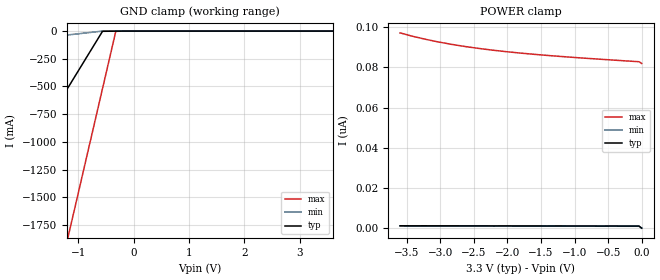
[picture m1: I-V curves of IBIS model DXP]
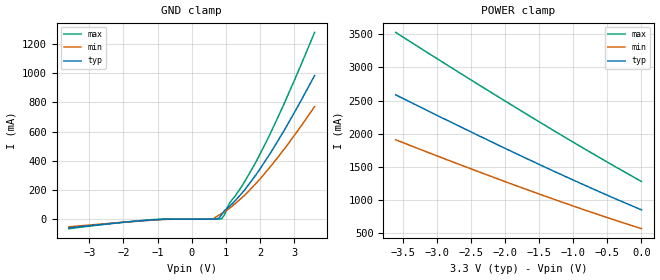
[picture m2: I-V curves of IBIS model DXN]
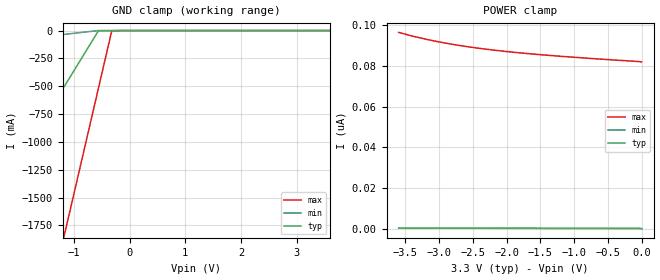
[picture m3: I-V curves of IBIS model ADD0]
| IBIS file MAX6654.ibs created at Maxim Integrated Products
[IBIS ver]   3.2
[File name]   max6654.ibs
[File Rev]   1.0
[Date]   February 19, 2010
[Source]   Data was acquired from HSpice simulations.
[Notes]   This is a microprocessor voltage monitor.
[Disclaimer] Maxim Integrated Products hereby grants the user of this
   IBIS model a non-exclusive, nontransferable license to use
   this IBIS model under the following terms. Before using
   this IBIS model, the user should read this license. If the
   user does not accept these terms, the IBIS model should be
   returned to Maxim Integrated Products within 30 days.
   The user is granted this license only to use the IBIS model
   and is not granted rights to sell, load, rent, lease or
   license the IBIS model in whole or in part, or in modified
   form to anyone other than user. User may modify the IBIS
   model to suit its specific applications but rights to
   derivative works and such modifications shall belong to
   Maxim Integrated Products. This IBIS model is provided on
   an "AS IS" basis and Maxim Integrated Products makes
   absolutely no warranty with respect to the information
   contained herein.MAXIM INTEGRATED PRODUCTS DISCLAIMS AND
   CUSTOMER WAIVES ALL WARRANTIES, EXPRESS OR IMPLIED,
   INCLUDING WARRANTIES OF MERCHANTABILITY OR FITNESS FOR A
   PARTICULAR PURPOSE. The entire risk as to quality and
   performance is with the Customer. ACCORDINGLY, IN NO EVENT
   SHALL THE COMPANY BE LIABLE FOR ANY DAMAGES, WHETHER IN
   CONTRACT OR TORT,INCLUDING ANY LOST PROFITS OR OTHER
   INCIDENTAL, CONSEQUENTIAL, EXEMPLARY, OR PUNITIVE DAMAGES
   ARISING OUT OF THE USE OR APPLICATION OF THE IBIS model
   provided in this package.Further, Maxim Integrated Products
   reserves the right to make changes without notice to any
   product herein to improve reliability, function, or design.
   Maxim Integrated Products does not convey any license under
   patent rights or any other intellectual property rights,
   including those of third parties.
   Maxim Integrated Products is not obligated to provide
   maintenance or support for the licensed IBIS model.
[Copyright]   Copyright of Maxim Integrated Products.
|   Component MAX6654
[Component]   MAX6654
[Manufacturer]   Maxim Integrated Products
[Package]
|variable   typ   min   max
R_pkg   0.052ohm   0.041ohm   0.065ohm
L_pkg   1.440nH   1.005nH   1.870nH
C_pkg   0.222pF   0.164pF   0.271pF
[Pin]  signal_name   model_name   R_pin   L_pin   C_pin
1   N.C   NC   NA   NA   NA
2   VCC   POWER   0.052   1.440nH   0.222pF
3   DXP   DXP   0.052   1.440nH   0.222pF
4   DXN   DXN   0.041   1.005nH   0.164pF
5   N.C   NC   NA   NA   NA
6   ADD1   ADD1   0.052   1.440nH   0.222pF
7   GND   GND   0.052   1.440nH   0.222pF
8   GND   GND   0.065   1.870nH   0.271pF
9   N.C   NC   NA   NA   NA
10   ADD0   ADD0   0.052   1.440nH   0.222pF
11   /ALERT\   ALERTB   0.052   1.440nH   0.222pF
12   SMBDATA   SMBDATA   0.041   1.005nH   0.164pF
13   N.C   NC   NA   NA   NA
14   SMBCLK   SMBCLK   0.052   1.440nH   0.222pF
15   /STBY\   STBYB   0.052   1.440nH   0.222pF
16   N.C   NC   NA   NA   NA
| Models and submodels in the file (8): DXP (Terminator), DXN (Terminator), ADD0 (Input), ADD1 (Input), SMBCLK (Input), STBYB (Input), ALERTB (Open_drain), SMBDATA (I/O_open_drain)
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|   DXP Input
[Model]   DXP
|Signals   DXP
Model_type   Terminator
C_comp   3.195E-12   2.653E-12   3.683E-12
[Temperature Range]   25   -55   125
[Voltage Range]   3.30V   3.00V   3.60V
[Pullup Reference]   3.30V   3.00V   3.60V
[Pulldown Reference]   0.00V   0.00V   0.00V
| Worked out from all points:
|   GND clamp passes 1 mA (typ) near -0.37 V on its own axis
[POWER_clamp]
| Note that the [POWER_clamp] voltage table is referenced to Vcc
| and is calculated using Vtable=Vcc - Vmeasured.
|V(V)   I(typ)   I(min)   I(max)
-3.6V     1.302nA    1.18nA     97.03nA
-3.4V     1.279nA    1.164nA    95.26nA
-3.24V    1.288nA    1.165nA    94.01nA
-3.04V    1.265nA    1.15nA     92.61nA
-2.84V    1.273nA    1.15nA     91.39nA
-2.72V    1.261nA    1.142nA    90.74nA
-2.36V    1.252nA    1.13nA     89.03nA
-2V       1.244nA    1.119nA    87.65nA
-1.44V    1.205nA    1.09nA     85.94nA
-840mV    1.206nA    1.077nA    84.46nA
-40mV     1.168nA    1.045nA    82.72nA
0V        129pA      112.7pA    81.88nA
[GND_clamp]
| Note that the [GND_clamp] voltage table is referenced to Gnd.
|V(V)   I(typ)   I(min)   I(max)
-3.6V     -2.483A    -169.4mA   -7.066A
-2.8V     -1.83A     -124.8mA   -5.343A
-2.72V    -1.765A    -120.3mA   -5.171A
-1.2V     -524.3mA   -35.66mA   -1.897A
-1.12V    -459mA     -31.2mA    -1.725A
-560mV    -1.93mA    -1.782uA   -519.1mA
-320mV    -772.1uA   -711.6nA   -2.201mA
3.6V      2.468nA    2.184nA    83.49nA
|   DXN Input
[Model]   DXN
|Signals   DXN
Model_type   Terminator
C_comp   0.484E-09   0.353E-09   0.676E-09
[Temperature Range]   25   -55   125
[Voltage Range]   3.30V   3.00V   3.60V
[Pullup Reference]   3.30V   3.00V   3.60V
[Pulldown Reference]   0.00V   0.00V   0.00V
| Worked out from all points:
|   GND clamp passes 1 mA (typ) near -0.79 V on its own axis
[POWER_clamp]
| Note that the [POWER_clamp] voltage table is referenced to Vcc
| and is calculated using Vtable=Vcc - Vmeasured.
|V(V)   I(typ)   I(min)   I(max)
-3.6V     2.586A     1.909A     3.525A
-2.64V    2.099A     1.527A     2.901A
-1.68V    1.625A     1.16A      2.293A
-920mV    1.266A     883.7mA    1.824A
0V        854mA      571.2mA    1.281A
[GND_clamp]
| Note that the [GND_clamp] voltage table is referenced to Gnd.
|V(V)   I(typ)   I(min)   I(max)
-3.6V     -60.67mA   -53.22mA   -65.81mA
-1.2V     -6.363mA   -8.032mA   -4.655mA
560mV     5.91uA     780.7uA    89.3uA
800mV     6.397mA    27.47mA    263.9uA
880mV     31.11mA    38.11mA    2.348mA
960mV     57.88mA    49.7mA     28.97mA
1.12V     90.13mA    76.22mA    114.1mA
1.52V     190.7mA    157.1mA    245mA
1.84V     290.7mA    234mA      373.1mA
2.24V     429.5mA    341.4mA    556.2mA
2.72V     613mA      483.3mA    798.3mA
3.6V      985.2mA    771.8mA    1.281A
|   ADD0 Input
[Model]   ADD0
|Signals   ADD0
Model_type   Input
Vinl = 0.8V
Vinh = 2.2V
C_comp   3.180E-12   2.622E-12   3.678E-12
[Temperature Range]   25   -55   125
[Voltage Range]   3.30V   3.00V   3.60V
[Pullup Reference]   3.30V   3.00V   3.60V
[Pulldown Reference]   0.00V   0.00V   0.00V
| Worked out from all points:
|   GND clamp passes 1 mA (typ) near -0.37 V on its own axis
[POWER_clamp]
| Note that the [POWER_clamp] voltage table is referenced to Vcc
| and is calculated using Vtable=Vcc - Vmeasured.
|V(V)   I(typ)   I(min)   I(max)
-3.6V     375.4pA    373.6pA    96.35nA
-3.44V    369.3pA    367.7pA    94.92nA
-3.28V    363pA      361.6pA    93.64nA
-3V       352.3pA    351.2pA    91.68nA
-2.84V    346.1pA    345.1pA    90.71nA
-2.64V    338.6pA    337.8pA    89.64nA
-2.28V    325pA      324.6pA    88.02nA
-1.8V     307.2pA    307.4pA    86.31nA
-1.36V    291.1pA    292pA      85.05nA
-840mV    272.6pA    274.4pA    83.78nA
-40mV     245.6pA    249.1pA    82.04nA
0V        142.7pA    129pA      81.88nA
[GND_clamp]
| Note that the [GND_clamp] voltage table is referenced to Gnd.
|V(V)   I(typ)   I(min)   I(max)
-3.6V     -2.483A    -169.4mA   -7.066A
-2.8V     -1.83A     -124.8mA   -5.343A
-2.72V    -1.765A    -120.3mA   -5.171A
-1.2V     -524.3mA   -35.66mA   -1.897A
-1.12V    -459mA     -31.2mA    -1.725A
-560mV    -1.93mA    -1.784uA   -519.1mA
-320mV    -772.1uA   -713.4nA   -2.201mA
3.6V      372.8pA    463.3pA    81.96nA
